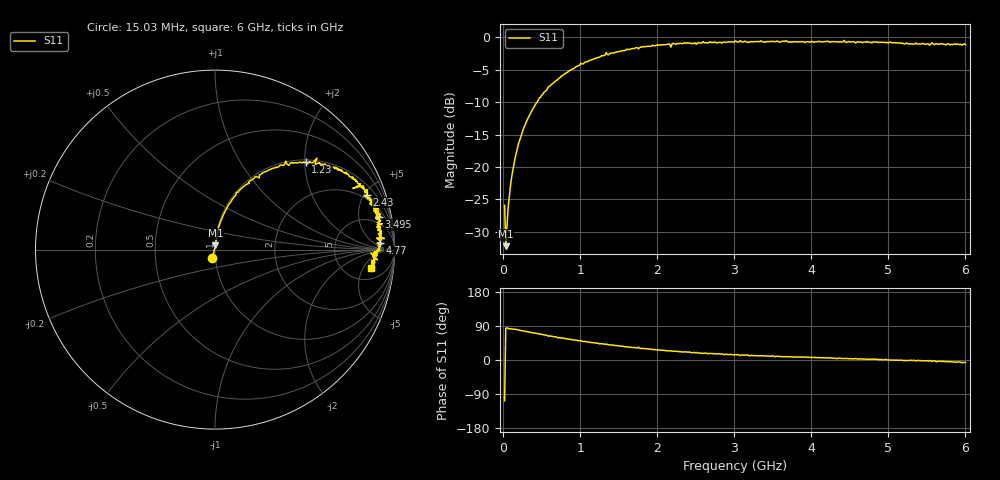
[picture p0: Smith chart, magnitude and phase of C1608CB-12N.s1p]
!	Network	Analyzer	HP8753E.07.74:	Oct	30	2002	Serial	No.	JP38451487
!	Hewlett-Packard
!	7	Sep	2009	9:35:38
!	Frequency	S11
#	HZ	S	RI	R	50
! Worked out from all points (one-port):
!   400 points, 15.03 MHz to 6 GHz, reference 50 ohm
!   lowest |S11| = -32.2 dB at 30.03 MHz (marker M1), VSWR 1.05, Z = 50.2 + j2.45 ohm
!   |S11| at or under -10 dB: start of sweep to 435.7 MHz
!   S11 on the Smith chart (normalised r, x): 15.03 MHz: 0.97, -0.09; 1.23 GHz: 1.06, +2.02; 2.43 GHz: 1.62, +5.22; 3.495 GHz: 3.21, +9.02; 4.77 GHz: 19, +9; 6 GHz: 9, -8
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1.502992e7  -0.0154 -0.0482
3.002985e7  0.00262 0.0244
6.00297e7  0.00533 0.0476
1.050295e8  0.0114 0.0815
1.95029e8  0.0282 0.149
2.550287e8  0.0444 0.189
4.650277e8  0.12 0.319
7.650262e8  0.267 0.429
1.005025e9  0.394 0.493
1.230024e9  0.505 0.486
1.335023e9  0.568 0.51
1.515022e9  0.624 0.463
1.93502e9  0.771 0.402
2.145019e9  0.81 0.367
2.175019e9  0.768 0.341
2.205019e9  0.828 0.354
2.265019e9  0.829 0.346
2.430018e9  0.846 0.306
3.015015e9  0.911 0.227
3.165014e9  0.885 0.219
3.195014e9  0.896 0.174
3.495013e9  0.915 0.182
3.525012e9  0.913 0.14
3.765011e9  0.91 0.135
4.515007e9  0.92 0.0579
4.770006e9  0.917 0.0348
5.265004e9  0.89 -0.0202
6e9  0.871 -0.101
